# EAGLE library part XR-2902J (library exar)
MICROCONTROLLER
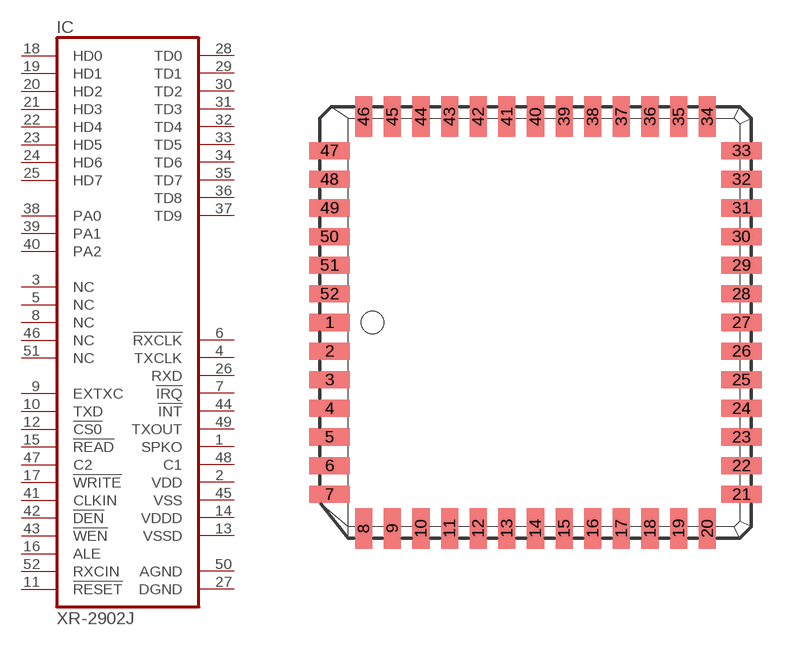
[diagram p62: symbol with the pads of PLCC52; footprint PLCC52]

Designator prefix IC

## XR-2902J (OC_FARNELL: unknown; OC_NEWARK: unknown)  [PLCC52]
1  SPKO  out
2  VDD  pwr
3  NC  nc
4  TXCLK  out
5  NC  nc
6  !RXCLK  out
7  !IRQ  out
8  NC  nc
9  EXTXC  in
10  TXD  in
11  !RESET  in
12  !CS0  in
13  VSSD  pwr
14  VDDD  pwr
15  !READ  in
16  ALE  in
17  !WRITE  in
18  HD0
19  HD1
20  HD2
21  HD3
22  HD4
23  HD5
24  HD6
25  HD7
26  RXD  out
27  DGND  pwr
28  TD0
29  TD1
30  TD2
31  TD3
32  TD4
33  TD5
34  TD6
35  TD7
36  TD8
37  TD9
38  PA0
39  PA1
40  PA2
41  CLKIN  in
42  !DEN  in
43  !WEN  in
44  !INT  out
45  VSS  pwr
46  NC  nc
47  C2  in
48  C1  out
49  TXOUT  out
50  AGND  pwr
51  NC  nc
52  RXCIN  in

## Footprint PLCC52 (pad centres in mm)
Plastic Leaded Chip Carrier
smd 1.8 x 0.76: 1 -9.13,0; 2 -9.13,-1.27; 3 -9.13,-2.54; 4 -9.13,-3.81; 5 -9.13,-5.08; 6 -9.13,-6.35; 7 -9.13,-7.62; 21 9.13,-7.62; 22 9.13,-6.35; 23 9.13,-5.08; 24 9.13,-3.81; 25 9.13,-2.54; 26 9.13,-1.27; 27 9.13,0; 28 9.13,1.27; 29 9.13,2.54; 30 9.13,3.81; 31 9.13,5.08; 32 9.13,6.35; 33 9.13,7.62; 47 -9.13,7.62; 48 -9.13,6.35; 49 -9.13,5.08; 50 -9.13,3.81; 51 -9.13,2.54; 52 -9.13,1.27
smd 0.76 x 1.8: 8 -7.62,-9.13; 9 -6.35,-9.13; 10 -5.08,-9.13; 11 -3.81,-9.13; 12 -2.54,-9.13; 13 -1.27,-9.13; 14 0,-9.13; 15 1.27,-9.13; 16 2.54,-9.13; 17 3.81,-9.13; 18 5.08,-9.13; 19 6.35,-9.13; 20 7.62,-9.13; 34 7.62,9.13; 35 6.35,9.13; 36 5.08,9.13; 37 3.81,9.13; 38 2.54,9.13; 39 1.27,9.13; 40 0,9.13; 41 -1.27,9.13; 42 -2.54,9.13; 43 -3.81,9.13; 44 -5.08,9.13; 45 -6.35,9.13; 46 -7.62,9.13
